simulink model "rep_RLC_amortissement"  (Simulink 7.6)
settings: Solver=ode15s  StartTime=0.0  StopTime=0.003  RelTol=1e-3
InitFcn:
  | L=1e-6;
  | C=1e-3;
  | 
  | z=0;
  | R=2*z*sqrt(L/C);
  | hold on
StopFcn:
  | clc
  | load second_ordre.mat
  | plot(x(1,:),x(2,:),x(1,:),x(3,:))
  | title('réponse d''un 2nd ordre avec dzeta=0')
  | grid
  | axis([0 1.5e-3 0 2])
  | xlabel('temps')
libraries: fl_lib x6, nesl_utility x4

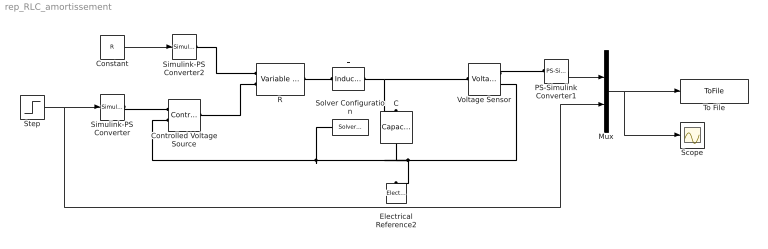
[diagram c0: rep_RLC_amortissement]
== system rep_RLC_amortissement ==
  C : fl_lib/Electrical/Electrical Elements/Capacitor  DialogController=NetworkEngine.DynNeDlgSource  SystemSampleTime=-1  c=C F  v0=0 V  r=1e-22 Ohm  g=0 1/Ohm  i_Log=off  v_Log=off  vc_Log=off  LocalVarNames=|i|v|vc  LocalVarDescs=|i|v|Internal variable for voltage across capacitor term  LocalVarLogging=[0 0 0]
  Constant : Constant  Value=R
  Controlled Voltage Source : fl_lib/Electrical/Electrical Sources/Controlled Voltage Source  DialogController=NetworkEngine.DynNeDlgSource  SystemSampleTime=-1  i_Log=off  v_Log=off  LocalVarNames=|i|v  LocalVarDescs=|i|v  LocalVarLogging=[0 0]
  Electrical Reference2 : fl_lib/Electrical/Electrical Elements/Electrical Reference  DialogController=NetworkEngine.DynNeDlgSource  SystemSampleTime=-1  i_Log=off  LocalVarNames=|i  LocalVarDescs=|i  LocalVarLogging=[]
  L : fl_lib/Electrical/Electrical Elements/Inductor  DialogController=NetworkEngine.DynNeDlgSource  SystemSampleTime=-1  l=L H  i0=0 A  r=0 Ohm  g=1e-22 1/Ohm  i_Log=off  v_Log=off  i_L_Log=off  LocalVarNames=|i|v|i_L  LocalVarDescs=|i|v|Internal variable for current through inductor term  LocalVarLogging=[0 0 0]
  Mux : Mux  Inputs=2
  PS-Simulink Converter1 : nesl_utility/PS-Simulink Converter  DialogController=NetworkEngine.DynNeUtilDlgSource  SystemSampleTime=-1  PhysicalDomain=network_engine_domain  LeftPortType=input  RightPortType=output  SubClassName=ps_output  Unit=1  AffineConversion=off
  R : fl_lib/Electrical/Electrical Elements/Variable Resistor  DialogController=NetworkEngine.DynNeDlgSource  SystemSampleTime=-1  Rmin=0 Ohm  i_Log=off  v_Log=off  LocalVarNames=|i|v  LocalVarDescs=|i|v  LocalVarLogging=[0 0]
  Scope : Scope
  Simulink-PS Converter : nesl_utility/Simulink-PS Converter  DialogController=NetworkEngine.DynNeUtilDlgSource  SystemSampleTime=-1  PhysicalDomain=network_engine_domain  LeftPortType=input  RightPortType=output  SubClassName=ps_input  Unit=1  AffineConversion=off  InputFilterTimeConstant=.001  UdotUserProvided=0
  Simulink-PS Converter2 : nesl_utility/Simulink-PS Converter  DialogController=NetworkEngine.DynNeUtilDlgSource  SystemSampleTime=-1  PhysicalDomain=network_engine_domain  LeftPortType=input  RightPortType=output  SubClassName=ps_input  Unit=1  AffineConversion=off  InputFilterTimeConstant=.001  UdotUserProvided=0
  Solver Configuration : nesl_utility/Solver Configuration  DialogController=NetworkEngine.DynNeUtilDlgSource  SystemSampleTime=-1  PhysicalDomain=network_engine_domain  LeftPortType=input  RightPortType=generic  SubClassName=solver  Accelerate=off  Profile=off  ResidualTolerance=1e-9  MaxNonlinIter=12  MaxModeIter=2  DoFixedCost=off  UseLocalSampling=off  DoDC=off  LinearAlgebra=Sparse  LocalSolverSampleTime=.001  LocalSolverChoice=NE_BACKWARD_EULER_ADVANCER  UseLocalSolver=off
  Step : Step  Time=0.5e-3  SampleTime=0
  To File : ToFile  Filename=second_ordre  MatrixName=x
  Voltage Sensor : fl_lib/Electrical/Electrical Sensors/Voltage Sensor  DialogController=NetworkEngine.DynNeDlgSource  SystemSampleTime=-1  i1_Log=off  v1_Log=off  LocalVarNames=|i1|v1  LocalVarDescs=|i1|v1  LocalVarLogging=[0 0]
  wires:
  Step/1 -> Simulink-PS Converter/1, Mux/2
  Constant/1 -> Simulink-PS Converter2/1
  PS-Simulink Converter1/1 -> Mux/1
  Mux/1 -> To File/1, Scope/1
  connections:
  L/LConn1 -- C/RConn1 -- Voltage Sensor/LConn1
  Controlled Voltage Source/RConn2 -- C/LConn1 -- Electrical Reference2/LConn1 -- Voltage Sensor/RConn2 -- Solver Configuration/RConn1
  R/RConn1 -- L/RConn1
  Voltage Sensor/RConn1 -- PS-Simulink Converter1/LConn1
  Simulink-PS Converter2/RConn1 -- R/LConn1
  Simulink-PS Converter/RConn1 -- Controlled Voltage Source/RConn1
  R/LConn2 -- Controlled Voltage Source/LConn1
